(* Logix 5000 DataType export Segment_Status; software revision 20.04 *)

TYPE Segment_Status :
STRUCT
   Speed_pulse_status : BOOL; {access Read Only}
   Exists : BOOL; {access Read Only}
   Group_number : INT; {access Read Only}
END_STRUCT
END_TYPE
